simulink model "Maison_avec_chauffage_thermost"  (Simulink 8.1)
settings: Solver=ode15s  SolverMode=SingleTasking  StartTime=0.0  StopTime=24*3600*10  FixedStep=1  MaxStep=10  RelTol=1e-3
InitFcn:
  | %   Simscape Demo "House Heating System"
  | max_temp = 23;    % Maximum temperature
  | min_temp = 18;     % Minimum temperature
  | % Walls
  | % House length = 30 m
  | lenHouse = 30;
  | % House width = 10 m
  | widHouse = 10;
  | % House height = 4 m
  | htHouse = 4;
  | wallArea = 2*lenHouse*htHouse + 2*widHouse*htHouse;
  | LWall = .2;
  | wallVolume = wallArea * LWall;
  | wallDensity = 1920;     % kg/m^3
  | wallMass = wallVolume * wallDensity;
  | c_wall = 835;           % J/kg/K
  | kWall = 0.038;  % Thermal conductivity [W/m/K]
  | % -------------------------------
  | % Windows
  | % Number of windows = 6
  | numWindows = 6;
  | % Height of windows = 1 m
  | htWindows = 1;
  | % Width of windows = 1 m
  | widWindows = 1;
  | windowArea = numWindows*htWindows*widWindows;
  | LWindow = .01;
  | windowVolume = windowArea * LWindow;
  | windowDensity = 2700;       % kg/m^3
  | windowMass = windowVolume * windowDensity;
  | c_window = 840;             % J/kg/K
  | kWindow = 0.78;             % Thermal conductivity [W/m/K]
  | % -------------------------------
  | % Roof
  | % Roof pitch = 40 deg
  | pitRoof = 40/180/pi;
  | roofArea =  2*(1/cos(pitRoof/2))*widHouse*lenHouse + tan(pitRoof)*widHouse;
  | LRoof = 0.2;
  | roofVolume = roofArea * LRoof;
  | roofDensity = 32;           % Glass fiber
  | roofMass = roofVolume * roofDensity;
  | kRoof = 0.038;              % Thermal conductivity [W/m/K]
  | c_roof = 835;               % J/kg/K
  | % -------------------------------
  | % Convective heat gransfer coefficients (W/M^2/K)
  | h_A_W = 24;         % Air-wall
  | h_W_Atm = 34;       % Wall-atmosphere
  | h_A_Wnd = 25;       % Air-window
  | h_Wnd_Atm = 32;     % Window-atmosphere
  | h_A_R = 12;         % Air-roof
  | h_R_Atm = 38;       % Roof-atmosphere
  | % -------------------------------
  | %Air
  | % Density of air at sea level = 1.2250 kg/m^3
  | densAir = 1.2250;
  | % Air mass inside the house
  | M_air = (lenHouse*widHouse*htHouse+tan(pitRoof)*widHouse*lenHouse)*densAir;
  | c_air = 1005.4;         % cp of air at 273 K [J/(kg*K]
  | % -------------------------------
  | % Heater
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model workspace: external: MATLAB Code (data not in the file)
libraries: fl_lib x31, nesl_utility x10

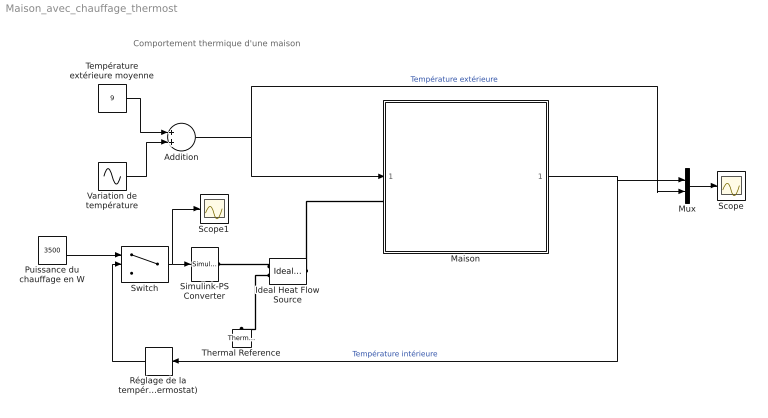
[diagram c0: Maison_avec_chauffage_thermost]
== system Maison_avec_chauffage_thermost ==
  note: Comportement thermique d'une maison
  Addition : Sum
  Ideal Heat Flow Source : fl_lib/Thermal/Thermal Sources/Ideal Heat Flow Source  Q_Log=off  T_Log=off  LocalVarNames=|Q|T  LocalVarDescs=|Q|T  LocalVarLogging=[0 0]
  Maison : Subsystem
  Mux : Mux  Inputs=2
  Puissance du chauffage en W : Constant  Value=3500
  Réglage de la température de consigne (thermostat) : Relay  OnSwitchValue=20  OffSwitchValue=19.9  OnOutputValue=0  OffOutputValue=1
  Scope : Scope
  Scope1 : Scope
  Simulink-PS Converter : nesl_utility/Simulink-PS Converter  PhysicalDomain=network_engine_domain  SubClassName=ps_input  LeftPortType=input  RightPortType=output  PseudoPeriodic=off  Frequencies=[]  NoiseDistribution=none  NoiseParameters=[]  Unit=J/s  AffineConversion=off  InputFiltering=off  SimscapeFilterOrder=1  InputFilterTimeConstant=0.001  UdotUserProvided=1
  Switch : Switch  Criteria=u2 > Threshold
  Température extérieure moyenne : Constant  Value=9
  Thermal Reference : fl_lib/Thermal/Thermal Elements/Thermal Reference  Q_Log=off  LocalVarNames=|Q  LocalVarDescs=|Q  LocalVarLogging=0
  Variation de température : Sin  Amplitude=3  Frequency=2*pi/(24*3600)  SampleTime=0
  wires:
  Température extérieure moyenne/1 -> Addition/1
  Variation de température/1 -> Addition/2
  Addition/1 -> Maison/1(Outdoor Temp), Mux/2  "Température extérieure"
  Maison/1(Room Temp Troom) -> Réglage de la température de consigne (thermostat)/1, Mux/1  "Température intérieure"
  Mux/1 -> Scope/1
  Switch/1 -> Simulink-PS Converter/1, Scope1/1
  Puissance du chauffage en W/1 -> Switch/1
  Réglage de la température de consigne (thermostat)/1 -> Switch/2
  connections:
  Ideal Heat Flow Source/LConn1 -- Maison/LConn1
  Ideal Heat Flow Source/RConn1 -- Simulink-PS Converter/RConn1
  Ideal Heat Flow Source/RConn2 -- Thermal Reference/LConn1

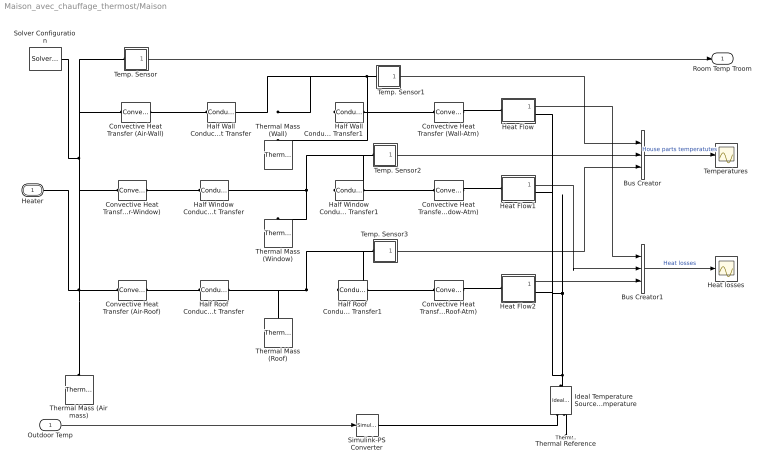
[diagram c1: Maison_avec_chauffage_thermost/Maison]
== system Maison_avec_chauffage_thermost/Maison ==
  Outdoor Temp : Inport
  Bus Creator : BusCreator  Inputs=3
  Bus Creator1 : BusCreator  Inputs=3
  Convective Heat Transfer (Air-Roof) : fl_lib/Thermal/Thermal Elements/Convective Heat Transfer  area=roofArea m^2  heat_tr_coeff=h_A_R W/m^2/K  Q_Log=off  T_Log=off  LocalVarNames=|heat_flow|temperature_diff  LocalVarDescs=|Heat flow (J/s)|Temperature difference (K)  LocalVarLogging=[0 0]
  Convective Heat Transfer (Air-Wall) : fl_lib/Thermal/Thermal Elements/Convective Heat Transfer  area=wallArea m^2  heat_tr_coeff=h_A_W W/m^2/K  Q_Log=off  T_Log=off  LocalVarNames=|heat_flow|temperature_diff  LocalVarDescs=|Heat flow (J/s)|Temperature difference (K)  LocalVarLogging=[0 0]
  Convective Heat Transfer (Roof-Atm) : fl_lib/Thermal/Thermal Elements/Convective Heat Transfer  area=roofArea m^2  heat_tr_coeff=h_R_Atm W/m^2/K  Q_Log=off  T_Log=off  LocalVarNames=|heat_flow|temperature_diff  LocalVarDescs=|Heat flow (J/s)|Temperature difference (K)  LocalVarLogging=[0 0]
  Convective Heat Transfer (Wall-Atm) : fl_lib/Thermal/Thermal Elements/Convective Heat Transfer  area=wallArea m^2  heat_tr_coeff=h_W_Atm W/m^2/K  Q_Log=off  T_Log=off  LocalVarNames=|heat_flow|temperature_diff  LocalVarDescs=|Heat flow (J/s)|Temperature difference (K)  LocalVarLogging=[0 0]
  Convective Heat Transfer (Window-Atm) : fl_lib/Thermal/Thermal Elements/Convective Heat Transfer  area=windowArea m^2  heat_tr_coeff=h_Wnd_Atm W/m^2/K  Q_Log=off  T_Log=off  LocalVarNames=|heat_flow|temperature_diff  LocalVarDescs=|Heat flow (J/s)|Temperature difference (K)  LocalVarLogging=[0 0]
  Convective Heat Transfer IAir-Window) : fl_lib/Thermal/Thermal Elements/Convective Heat Transfer  area=windowArea m^2  heat_tr_coeff=h_A_Wnd W/m^2/K  Q_Log=off  T_Log=off  LocalVarNames=|heat_flow|temperature_diff  LocalVarDescs=|Heat flow (J/s)|Temperature difference (K)  LocalVarLogging=[0 0]
  Half Roof Conductive Heat Transfer : fl_lib/Thermal/Thermal Elements/Conductive Heat Transfer  area=roofArea m^2  thickness=LRoof/2 m  th_cond=kRoof W/m/K  Q_Log=off  T_Log=off  LocalVarNames=|heat_flow|temperature_diff  LocalVarDescs=|Heat flow (J/s)|Temperature difference (K)  LocalVarLogging=[0 0]
  Half Roof Conductive Heat Transfer1 : fl_lib/Thermal/Thermal Elements/Conductive Heat Transfer  area=roofArea m^2  thickness=LRoof/2 m  th_cond=kRoof W/m/K  Q_Log=off  T_Log=off  LocalVarNames=|heat_flow|temperature_diff  LocalVarDescs=|Heat flow (J/s)|Temperature difference (K)  LocalVarLogging=[0 0]
  Half Wall Conductive Heat Transfer : fl_lib/Thermal/Thermal Elements/Conductive Heat Transfer  area=wallArea m^2  thickness=LWall/2 m  th_cond=kWall W/m/K  Q_Log=off  T_Log=off  LocalVarNames=|heat_flow|temperature_diff  LocalVarDescs=|Heat flow (J/s)|Temperature difference (K)  LocalVarLogging=[0 0]
  Half Wall Conductive Heat Transfer1 : fl_lib/Thermal/Thermal Elements/Conductive Heat Transfer  area=wallArea m^2  thickness=LWall/2 m  th_cond=kWall W/m/K  Q_Log=off  T_Log=off  LocalVarNames=|heat_flow|temperature_diff  LocalVarDescs=|Heat flow (J/s)|Temperature difference (K)  LocalVarLogging=[0 0]
  Half Window Conductive Heat Transfer : fl_lib/Thermal/Thermal Elements/Conductive Heat Transfer  area=windowArea m^2  thickness=LWindow/2 m  th_cond=kWindow W/m/K  Q_Log=off  T_Log=off  LocalVarNames=|heat_flow|temperature_diff  LocalVarDescs=|Heat flow (J/s)|Temperature difference (K)  LocalVarLogging=[0 0]
  Half Window Conductive Heat Transfer1 : fl_lib/Thermal/Thermal Elements/Conductive Heat Transfer  area=windowArea m^2  thickness=LWindow/2 m  th_cond=kWindow W/m/K  Q_Log=off  T_Log=off  LocalVarNames=|heat_flow|temperature_diff  LocalVarDescs=|Heat flow (J/s)|Temperature difference (K)  LocalVarLogging=[0 0]
  Heat Flow : Subsystem
  Heat Flow1 : Subsystem
  Heat Flow2 : Subsystem
  Heat losses : Scope
  Ideal Temperature Source. Outdoor temperature : fl_lib/Thermal/Thermal Sources/Ideal Temperature Source  Q_Log=off  T_Log=off  LocalVarNames=|heat_flow|T_differential  LocalVarDescs=|Heat flow rate through the source (J/s)|Temperature differential across the source (K)  LocalVarLogging=[0 0]
  Simulink-PS Converter : nesl_utility/Simulink-PS Converter  PhysicalDomain=network_engine_domain  SubClassName=ps_input  LeftPortType=input  RightPortType=output  PseudoPeriodic=off  Frequencies=[]  NoiseDistribution=none  NoiseParameters=[]  Unit=C  AffineConversion=on  InputFiltering=off  SimscapeFilterOrder=1  InputFilterTimeConstant=.001  UdotUserProvided=1
  Solver Configuration : nesl_utility/Solver Configuration  PhysicalDomain=network_engine_domain  SubClassName=solver  LeftPortType=input  RightPortType=generic  Accelerate=off  Tones=[]  Harmonics=[]  SimulateNoise=off  Profile=off  UseLocalSampling=off  EnableSwitchedLinearOptims=on  FrequencyDomain=off  UseCCode=off  UseNewInitialization=off  DoDC=off  ResidualTolerance=1e-9  UseLocalSolver=off  LocalSolverChoice=NE_BACKWARD_EULER_ADVANCER  LocalSolverSampleTime=.001  DoFixedCost=off  MaxNonlinIter=3  MaxModeIter=2  LinearAlgebra=Sparse  DelaysMemoryBudget=1024
  Temp. Sensor : Subsystem
  Temp. Sensor1 : Subsystem
  Temp. Sensor2 : Subsystem
  Temp. Sensor3 : Subsystem
  Temperatures : Scope
  Thermal Mass (Air mass) : fl_lib/Thermal/Thermal Elements/Thermal Mass  mass=M_air kg  sp_heat=c_air J/kg/K  init_temp=TinIC C  Q_Log=off  LocalVarNames=|heat_flow|temperature  LocalVarDescs=|Heat flow (J/s)|Mass temperature (K)  LocalVarLogging=[0 0]
  Thermal Mass (Roof) : fl_lib/Thermal/Thermal Elements/Thermal Mass  mass=roofMass kg  sp_heat=c_roof J/kg/K  init_temp=TinIC C  Q_Log=off  LocalVarNames=|heat_flow|temperature  LocalVarDescs=|Heat flow (J/s)|Mass temperature (K)  LocalVarLogging=[0 0]
  Thermal Mass (Wall) : fl_lib/Thermal/Thermal Elements/Thermal Mass  mass=wallMass kg  sp_heat=c_wall J/kg/K  init_temp=TinIC C  Q_Log=off  LocalVarNames=|heat_flow|temperature  LocalVarDescs=|Heat flow (J/s)|Mass temperature (K)  LocalVarLogging=[0 0]
  Thermal Mass (Window) : fl_lib/Thermal/Thermal Elements/Thermal Mass  mass=windowMass kg  sp_heat=c_window J/kg/K  init_temp=TinIC C  Q_Log=off  LocalVarNames=|heat_flow|temperature  LocalVarDescs=|Heat flow (J/s)|Mass temperature (K)  LocalVarLogging=[0 0]
  Thermal Reference : fl_lib/Thermal/Thermal Elements/Thermal Reference  Q_Log=off  LocalVarNames=|Q  LocalVarDescs=|Q  LocalVarLogging=[]
  Heater : PMIOPort  Tag=PMCPort  Port=1  Side=Left
  Room Temp Troom : Outport  InitialOutput=0
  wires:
  Outdoor Temp/1 -> Simulink-PS Converter/1
  Temp. Sensor/1(T) -> Room Temp Troom/1
  Temp. Sensor1/1(T) -> Bus Creator/1
  Temp. Sensor2/1(T) -> Bus Creator/2
  Temp. Sensor3/1(T) -> Bus Creator/3
  Bus Creator/1 -> Temperatures/1  "House parts temperatutes"
  Heat Flow2/1(Q) -> Bus Creator1/3
  Heat Flow1/1(Q) -> Bus Creator1/2
  Heat Flow/1(Q) -> Bus Creator1/1
  Bus Creator1/1 -> Heat losses/1  "Heat losses"
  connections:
  Thermal Reference/LConn1 -- Ideal Temperature Source. Outdoor temperature/RConn2
  Ideal Temperature Source. Outdoor temperature/RConn1 -- Simulink-PS Converter/RConn1
  Thermal Mass (Air mass)/LConn1 -- Heater/RConn1 -- Temp. Sensor/LConn1 -- Solver Configuration/RConn1 -- Convective Heat Transfer (Air-Wall)/LConn1 -- Convective Heat Transfer IAir-Window)/LConn1 -- Convective Heat Transfer (Air-Roof)/LConn1
  Convective Heat Transfer (Air-Wall)/RConn1 -- Half Wall Conductive Heat Transfer/LConn1
  Temp. Sensor1/LConn1 -- Half Wall Conductive Heat Transfer/RConn1 -- Thermal Mass (Wall)/LConn1 -- Half Wall Conductive Heat Transfer1/LConn1
  Half Wall Conductive Heat Transfer1/RConn1 -- Convective Heat Transfer (Wall-Atm)/LConn1
  Convective Heat Transfer IAir-Window)/RConn1 -- Half Window Conductive Heat Transfer/LConn1
  Temp. Sensor2/LConn1 -- Half Window Conductive Heat Transfer/RConn1 -- Thermal Mass (Window)/LConn1 -- Half Window Conductive Heat Transfer1/LConn1
  Half Window Conductive Heat Transfer1/RConn1 -- Convective Heat Transfer (Window-Atm)/LConn1
  Convective Heat Transfer (Air-Roof)/RConn1 -- Half Roof Conductive Heat Transfer/LConn1
  Temp. Sensor3/LConn1 -- Thermal Mass (Roof)/LConn1 -- Half Roof Conductive Heat Transfer/RConn1 -- Half Roof Conductive Heat Transfer1/LConn1
  Half Roof Conductive Heat Transfer1/RConn1 -- Convective Heat Transfer (Roof-Atm)/LConn1
  Convective Heat Transfer (Wall-Atm)/RConn1 -- Heat Flow/LConn1
  Convective Heat Transfer (Window-Atm)/RConn1 -- Heat Flow1/LConn1
  Convective Heat Transfer (Roof-Atm)/RConn1 -- Heat Flow2/LConn1
  Ideal Temperature Source. Outdoor temperature/LConn1 -- Heat Flow/RConn1 -- Heat Flow1/RConn1 -- Heat Flow2/RConn1

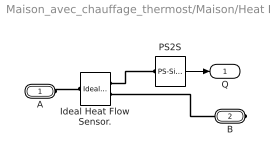
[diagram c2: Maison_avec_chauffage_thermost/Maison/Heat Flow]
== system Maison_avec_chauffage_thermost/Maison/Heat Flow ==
  Ideal Heat Flow Sensor. : fl_lib/Thermal/Thermal Sensors/Ideal Heat Flow Sensor  Q_Log=off  T_Log=off  LocalVarNames=|Q|T  LocalVarDescs=|Q|T  LocalVarLogging=[]
  PS2S : nesl_utility/PS-Simulink Converter  PhysicalDomain=network_engine_domain  SubClassName=ps_output  LeftPortType=input  RightPortType=output  PseudoPeriodic=off  Frequencies=[]  Unit=1  AffineConversion=off
  A : PMIOPort  Port=1  Side=Left
  B : PMIOPort  Port=2  Side=Right
  Q : Outport
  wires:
  PS2S/1 -> Q/1
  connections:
  Ideal Heat Flow Sensor./RConn1 -- PS2S/LConn1
  A/RConn1 -- Ideal Heat Flow Sensor./LConn1
  B/RConn1 -- Ideal Heat Flow Sensor./RConn2

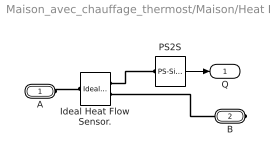
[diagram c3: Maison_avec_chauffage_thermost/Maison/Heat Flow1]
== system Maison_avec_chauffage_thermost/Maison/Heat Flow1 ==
  Ideal Heat Flow Sensor. : fl_lib/Thermal/Thermal Sensors/Ideal Heat Flow Sensor  Q_Log=off  T_Log=off  LocalVarNames=|Q|T  LocalVarDescs=|Q|T  LocalVarLogging=[]
  PS2S : nesl_utility/PS-Simulink Converter  PhysicalDomain=network_engine_domain  SubClassName=ps_output  LeftPortType=input  RightPortType=output  PseudoPeriodic=off  Frequencies=[]  Unit=1  AffineConversion=off
  A : PMIOPort  Port=1  Side=Left
  B : PMIOPort  Port=2  Side=Right
  Q : Outport
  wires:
  PS2S/1 -> Q/1
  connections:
  B/RConn1 -- Ideal Heat Flow Sensor./RConn2
  A/RConn1 -- Ideal Heat Flow Sensor./LConn1
  Ideal Heat Flow Sensor./RConn1 -- PS2S/LConn1

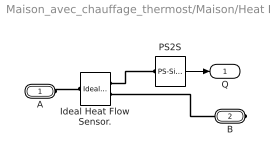
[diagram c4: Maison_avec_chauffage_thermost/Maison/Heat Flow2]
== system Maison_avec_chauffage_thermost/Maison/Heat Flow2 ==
  Ideal Heat Flow Sensor. : fl_lib/Thermal/Thermal Sensors/Ideal Heat Flow Sensor  Q_Log=off  T_Log=off  LocalVarNames=|Q|T  LocalVarDescs=|Q|T  LocalVarLogging=[]
  PS2S : nesl_utility/PS-Simulink Converter  PhysicalDomain=network_engine_domain  SubClassName=ps_output  LeftPortType=input  RightPortType=output  PseudoPeriodic=off  Frequencies=[]  Unit=1  AffineConversion=off
  A : PMIOPort  Port=1  Side=Left
  B : PMIOPort  Port=2  Side=Right
  Q : Outport
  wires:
  PS2S/1 -> Q/1
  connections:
  Ideal Heat Flow Sensor./RConn1 -- PS2S/LConn1
  A/RConn1 -- Ideal Heat Flow Sensor./LConn1
  B/RConn1 -- Ideal Heat Flow Sensor./RConn2

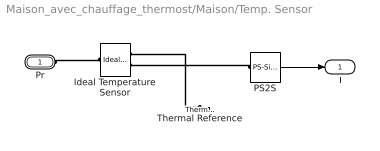
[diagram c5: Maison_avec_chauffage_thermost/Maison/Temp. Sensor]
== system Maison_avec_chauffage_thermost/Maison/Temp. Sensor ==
  Ideal Temperature Sensor : fl_lib/Thermal/Thermal Sensors/Ideal Temperature Sensor  Qs_Log=off  Ts_Log=off  LocalVarNames=|Qs|Ts  LocalVarDescs=|Qs|Ts  LocalVarLogging=[]
  PS2S : nesl_utility/PS-Simulink Converter  PhysicalDomain=network_engine_domain  SubClassName=ps_output  LeftPortType=input  RightPortType=output  PseudoPeriodic=off  Frequencies=[]  Unit=C  AffineConversion=on
  Thermal Reference : fl_lib/Thermal/Thermal Elements/Thermal Reference  Q_Log=off  LocalVarNames=|Q  LocalVarDescs=|Q  LocalVarLogging=[]
  Pr : PMIOPort  Port=1  Side=Left
  T : Outport
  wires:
  PS2S/1 -> T/1
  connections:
  Ideal Temperature Sensor/RConn1 -- Thermal Reference/LConn1
  PS2S/LConn1 -- Ideal Temperature Sensor/RConn2
  Pr/RConn1 -- Ideal Temperature Sensor/LConn1

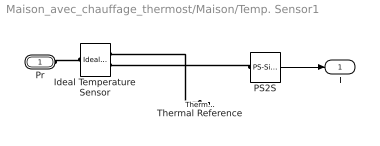
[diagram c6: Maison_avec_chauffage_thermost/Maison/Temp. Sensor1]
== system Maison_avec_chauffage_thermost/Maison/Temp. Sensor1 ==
  Ideal Temperature Sensor : fl_lib/Thermal/Thermal Sensors/Ideal Temperature Sensor  Qs_Log=off  Ts_Log=off  LocalVarNames=|Qs|Ts  LocalVarDescs=|Qs|Ts  LocalVarLogging=[]
  PS2S : nesl_utility/PS-Simulink Converter  PhysicalDomain=network_engine_domain  SubClassName=ps_output  LeftPortType=input  RightPortType=output  PseudoPeriodic=off  Frequencies=[]  Unit=C  AffineConversion=on
  Thermal Reference : fl_lib/Thermal/Thermal Elements/Thermal Reference  Q_Log=off  LocalVarNames=|Q  LocalVarDescs=|Q  LocalVarLogging=[]
  Pr : PMIOPort  Port=1  Side=Left
  T : Outport
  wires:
  PS2S/1 -> T/1
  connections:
  Pr/RConn1 -- Ideal Temperature Sensor/LConn1
  PS2S/LConn1 -- Ideal Temperature Sensor/RConn2
  Ideal Temperature Sensor/RConn1 -- Thermal Reference/LConn1

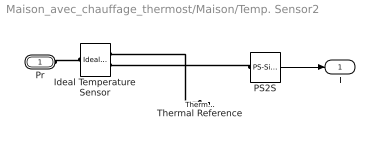
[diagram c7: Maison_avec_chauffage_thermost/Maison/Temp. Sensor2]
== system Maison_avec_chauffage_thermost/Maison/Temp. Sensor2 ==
  Ideal Temperature Sensor : fl_lib/Thermal/Thermal Sensors/Ideal Temperature Sensor  Qs_Log=off  Ts_Log=off  LocalVarNames=|Qs|Ts  LocalVarDescs=|Qs|Ts  LocalVarLogging=[]
  PS2S : nesl_utility/PS-Simulink Converter  PhysicalDomain=network_engine_domain  SubClassName=ps_output  LeftPortType=input  RightPortType=output  PseudoPeriodic=off  Frequencies=[]  Unit=C  AffineConversion=on
  Thermal Reference : fl_lib/Thermal/Thermal Elements/Thermal Reference  Q_Log=off  LocalVarNames=|Q  LocalVarDescs=|Q  LocalVarLogging=[]
  Pr : PMIOPort  Port=1  Side=Left
  T : Outport
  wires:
  PS2S/1 -> T/1
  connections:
  Ideal Temperature Sensor/RConn1 -- Thermal Reference/LConn1
  PS2S/LConn1 -- Ideal Temperature Sensor/RConn2
  Pr/RConn1 -- Ideal Temperature Sensor/LConn1

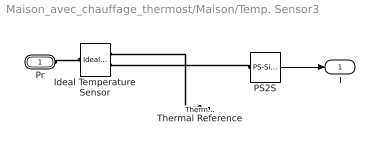
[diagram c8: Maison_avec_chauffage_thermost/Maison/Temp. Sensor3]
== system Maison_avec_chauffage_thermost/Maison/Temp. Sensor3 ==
  Ideal Temperature Sensor : fl_lib/Thermal/Thermal Sensors/Ideal Temperature Sensor  Qs_Log=off  Ts_Log=off  LocalVarNames=|Qs|Ts  LocalVarDescs=|Qs|Ts  LocalVarLogging=[]
  PS2S : nesl_utility/PS-Simulink Converter  PhysicalDomain=network_engine_domain  SubClassName=ps_output  LeftPortType=input  RightPortType=output  PseudoPeriodic=off  Frequencies=[]  Unit=C  AffineConversion=on
  Thermal Reference : fl_lib/Thermal/Thermal Elements/Thermal Reference  Q_Log=off  LocalVarNames=|Q  LocalVarDescs=|Q  LocalVarLogging=[]
  Pr : PMIOPort  Port=1  Side=Left
  T : Outport
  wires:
  PS2S/1 -> T/1
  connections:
  Pr/RConn1 -- Ideal Temperature Sensor/LConn1
  PS2S/LConn1 -- Ideal Temperature Sensor/RConn2
  Ideal Temperature Sensor/RConn1 -- Thermal Reference/LConn1
